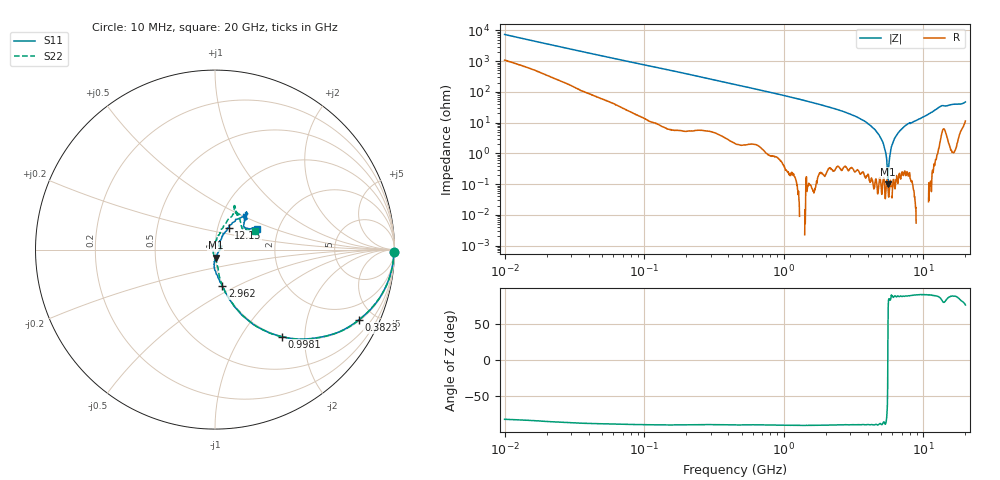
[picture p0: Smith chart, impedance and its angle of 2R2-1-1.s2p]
!Keysight Technologies,P5008B,MY61100088,A.16.20.02
!Date: Monday, May 27, 2024 14:26:51
!Correction: S11(C* 2-Port  )
!S21(C* 2-Port  )
!S12(C* 2-Port  )
!S22(C* 2-Port  )
!S2P File: Measurements: S11, S21, S12, S22:Log Frequency Sweep
# Hz S  dB  R 50
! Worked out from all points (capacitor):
!   1601 points, 10 MHz to 20 GHz, reference 50 ohm
!   read as one part in series: C = 2.18 pF near 10.39 MHz
!   lowest |Z| = 100 mohm at 5.572 GHz (marker M1)
!   series resonance near 5.563 GHz, so ESL is about 380 pH
!   S11 on the Smith chart (normalised r, x): 10 MHz: open; 382.3 MHz: 1.06, -4.04; 998.1 MHz: 1.00, -1.54; 2.962 GHz: 1.00, -0.42; 12.15 GHz: 1.13, +0.28; 20 GHz: 1.55, +0.38
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1e7  -0.00 -0.8  -37.39 80.8  -37.39 80.8  -0.02 -0.8
3.555162e7  -0.03 -2.7  -26.36 84.2  -26.36 84.2  -0.04 -2.8
1.263918e8  -0.15 -9.4  -15.82 79.8  -15.83 79.8  -0.14 -9.4
3.823237e8  -1.00 -26.1  -7.14 62.9  -7.15 62.9  -1.00 -26.3
4.472136e8  -1.29 -29.9  -6.11 59.4  -6.12 59.4  -1.28 -30.0
9.981281e8  -4.28 -52.5  -2.06 37.2  -2.07 37.2  -4.27 -52.6
1.589917e9  -7.54 -65.9  -0.84 24.0  -0.85 24.0  -7.50 -65.7
2.962417e9  -13.65 -78.7  -0.19 9.8  -0.20 9.9  -13.66 -78.5
4.332092e9  -19.88 -92.0  -0.04 2.2  -0.05 2.2  -20.21 -80.8
5.572426e9  -27.03 -85.8  0.01 -2.6  -0.01 -2.6  -26.90 -92.5
5.652411e9  -27.45 -86.9  0.00 -2.9  -0.01 -2.9  -27.36 -94.6
6.395515e9  -32.29 -47.5  0.02 -5.3  0.01 -5.3  -34.64 -117.7
6.867879e9  -32.41 -15.0  0.02 -6.8  0.01 -6.8  -36.99 -171.6
7.697294e9  -28.71 24.2  0.02 -9.2  0.01 -9.2  -31.66 120.7
8.344716e9  -30.06 21.0  0.03 -10.9  0.02 -10.9  -32.35 120.5
9.264046e9  -29.91 45.6  0.04 -13.3  0.02 -13.3  -29.97 98.1
1.023592e10  -26.10 60.8  0.03 -16.0  0.02 -16.0  -26.44 81.6
1.214507e10  -16.77 58.1  -0.08 -21.7  -0.09 -21.6  -17.13 70.0
1.361179e10  -12.20 46.5  -0.59 -25.7  -0.60 -25.6  -12.44 58.0
1.62275e10  -11.41 49.0  -0.34 -29.4  -0.35 -29.4  -11.62 65.1
1.862442e10  -13.76 36.1  -0.59 -35.4  -0.60 -35.4  -14.36 38.9
2e10  -11.76 26.3  -1.13 -38.4  -1.14 -38.4  -12.26 25.3
